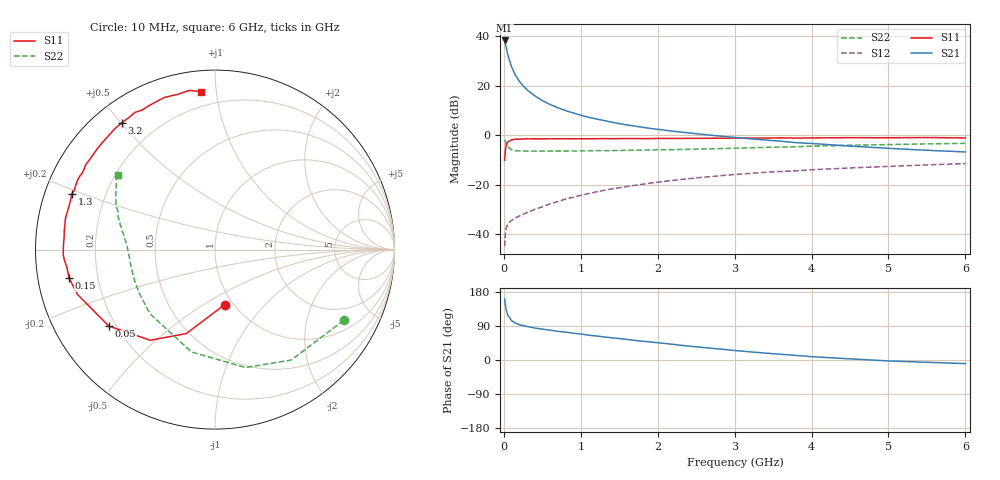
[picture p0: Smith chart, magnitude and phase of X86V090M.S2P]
! SIEMENS Small Signal Semiconductors
! BFP136W
! Si NPN RF Bipolar Junction Transistor in SOT343
! VCE = 6 V  IC = 90 mA
! Common Emitter S-Parameters:  September  1994
# GHz  S  MA  R  50
!  f  S11  S21  S12  S22
! GHz  MAG  ANG  MAG  ANG  MAG  ANG  MAG  ANG
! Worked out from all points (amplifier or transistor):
!   40 points, 10 MHz to 6 GHz, reference 50 ohm
!   highest |S21| = 38.3 dB at 10 MHz (marker M1)
!   |S21| within 3 dB of that: start of sweep to 32.11 MHz
!   unconditionally stable (mu >= 1): 567.1 MHz to 2.952 GHz
!   at 200 MHz: K = 0.64, MSG = 27.3 dB, |S12| = -32.7 dB
!   at 1.5 GHz: K = 1.10, MAG = 11.1 dB, |S12| = -21.2 dB
!   at 6 GHz: K = 0.97, MSG = 2.4 dB, |S12| = -11.5 dB
!   S11 on the Smith chart (normalised r, x): 10 MHz: 0.92, -0.62; 50 MHz: 0.17, -0.31; 150 MHz: 0.09, -0.10; 1.3 GHz: 0.08, +0.19; 3.2 GHz: 0.08, +0.50; 6 GHz: 0.11, +0.91
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0.01  0.3109 -79.8  82.68 160.7  0.0057 69.6  0.8185 -28.8
0.02  0.4947 -108.9  71.38 144.6  0.0101 57.9  0.7477 -55.4
0.03  0.6205 -125.5  60.61 133.0  0.013 49.6  0.6788 -75.5
0.05  0.7286 -144.2  43.53 118.7  0.016 39.9  0.585 -103.0
0.1  0.8058 -161.9  24.2 104.0  0.019 35.3  0.5089 -135.6
0.15  0.8285 -169.0  16.48 97.4  0.0211 37.8  0.4872 -149.4
0.2  0.831 -173.1  12.4 93.4  0.0232 39.3  0.4813 -156.9
0.25  0.8417 -176.2  9.997 90.6  0.0252 42.3  0.4794 -161.6
0.3  0.8464 -178.1  8.359 88.4  0.0271 45.0  0.4769 -164.9
0.4  0.8446 178.0  6.299 84.5  0.0315 49.3  0.4771 -169.2
0.5  0.8435 175.0  5.021 81.4  0.0357 52.3  0.4773 -172.1
0.6  0.8464 172.9  4.188 78.8  0.0407 54.9  0.4782 -174.0
0.7  0.8475 170.4  3.608 75.8  0.0455 56.7  0.4794 -175.4
0.9  0.8501 166.6  2.826 70.9  0.0556 58.4  0.4815 -178.0
1.1  0.849 162.2  2.31 65.6  0.0659 59.4  0.4849 -179.7
1.3  0.8558 158.6  1.988 60.9  0.0767 59.5  0.4882 178.6
1.7  0.8579 151.7  1.532 51.8  0.0968 57.8  0.4966 175.5
2.2  0.8599 143.3  1.207 41.3  0.1222 54.5  0.5108 171.9
3.2  0.8768 126.3  0.848 21.5  0.169 45.5  0.5557 163.3
4.5  0.8936 108.3  0.604 3.0  0.218 33.7  0.6266 152.0
5.5  0.8986 99.1  0.496 -6.0  0.2507 25.7  0.6691 145.3
6  0.8824 94.9  0.459 -9.5  0.267 21.5  0.6854 142.4
